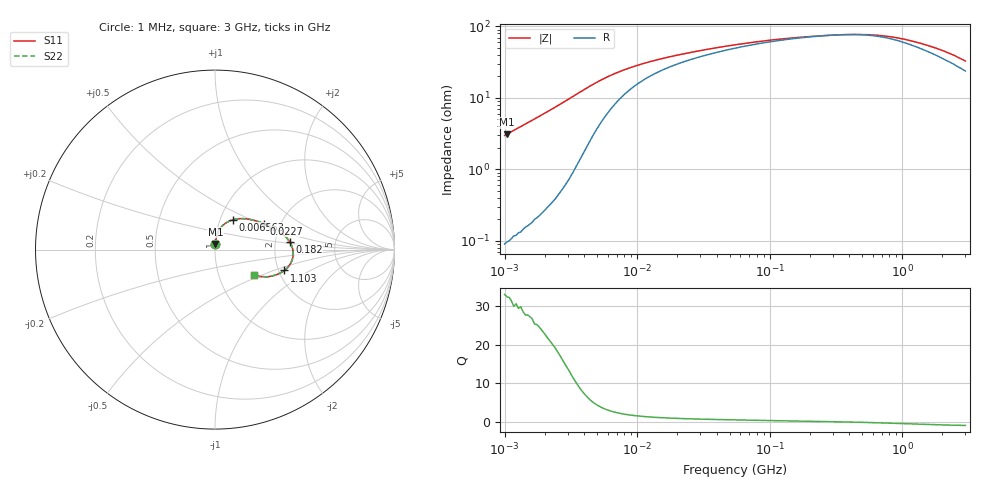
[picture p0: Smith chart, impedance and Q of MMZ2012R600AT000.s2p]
! S-parameter Generated by TDK Corporation
! Copyright(C) 2016 TDK Corporation.
! All Rights Reserved.
! TDK P/N: MMZ2012R600AT000 (Chip Beads)
! Property: |Z|=60¶ at 100MHz
! Size(LxWxT): 2x1.25x0.85mm, 0.079x0.049x0.033inches
! Model Type: s2p (Touchstone File Format Version 1.0)
! Frequency: DC=Yes Start=1MHz Stop=3000MHz 202points Log-sweep
! Note: This model was converted from impedance.
! Model Generated on May. 16, 2016
! Hash(MD5):
! Port Assignments:
!  1 ---@@@--- 2
! Applicable Conditions:
!  Temperature = 25 degC
!  DC Bias Current = 0 A
!  Small Signal Operation
! Terms and conditions regarding TDK Simulation Models
! (1)This simulation model is being provided solely for informational purposes. Please refer to the specifications of the products in terms of detailed characteristics of such products.
! (2)In no event shall TDK Corporation of any of its subsidiaries be liable for any loss or damage arising, directly or indirectly,
!  From any information contained in this simulation model, including, but not limited to loss or damages arising from any inaccuracies, omissions or errors in connection with such information.
! (3)Any and all copyrights on this simulation model are owned by TDK Corporation.
!  Duplication or redistribution of this simulation model without prior written permission from TDK Corporation is prohibited.
! (4)This simulation model is subject to any modification or change without any prior notice.
! (5)Neither TDK Corporation nor any of its subsidiaries shall make any warranty, express or implied,
!  Including but not limited to the correctness, implied warranties of merchantability and fitness for a particular purpose with respect to this simulation models.
! (6)The use of this simulation model shall be deemed to have consented to the terms and conditions hereof.
# MHz S MA R 50
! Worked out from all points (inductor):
!   201 points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, 1 MHz to 3 GHz, reference 50 ohm
!   read as one part in series: L = 477 nH near 1.041 MHz
!   highest Q = 32.5 at 1.041 MHz (marker M1), where L = 476 nH
!   self-resonance near 345.4 MHz
!   S11 on the Smith chart (normalised r, x): 1 MHz: 1.00, +0.06; 6.563 MHz: 1.15, +0.40; 22.7 MHz: 1.64, +0.53; 182 MHz: 2.40, +0.25; 1.103 GHz: 2.15, -0.60; 3 GHz: 1.48, -0.45
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1  0.02985 86.6  0.9987 -1.7  0.9987 -1.7  0.02985 86.6
1.040844  0.03111 86.5  0.9986 -1.8  0.9986 -1.8  0.03111 86.5
2.13957  0.06497 83.6  0.9949 -3.7  0.9949 -3.7  0.06497 83.6
3.067588  0.09602 80.2  0.9882 -5.5  0.9882 -5.5  0.09602 80.2
3.900413  0.1248 75.5  0.9762 -7.1  0.9762 -7.1  0.1248 75.5
5.161903  0.1633 67.0  0.9482 -9.1  0.9482 -9.1  0.1633 67.0
6.563319  0.1951 58.6  0.9138 -10.5  0.9138 -10.5  0.1951 58.6
9.410094  0.2357 47.0  0.8566 -11.6  0.8566 -11.6  0.2357 47.0
14.61624  0.2754 35.9  0.7937 -11.7  0.7937 -11.7  0.2754 35.9
22.70269  0.3086 28.0  0.7417 -11.2  0.7417 -11.2  0.3086 28.0
54.77226  0.3654 17.0  0.6592 -9.3  0.6592 -9.3  0.3654 17.0
99.84923  0.3956 11.2  0.6167 -7.2  0.6167 -7.2  0.3956 11.2
182.0241  0.418 6.0  0.5859 -4.3  0.5859 -4.3  0.418 6.0
213.6344  0.4228 4.6  0.5795 -3.3  0.5795 -3.3  0.4228 4.6
457.0858  0.4366 -3.2  0.5646 2.5  0.5646 2.5  0.4366 -3.2
604.9187  0.4346 -7.0  0.5711 5.3  0.5711 5.3  0.4346 -7.0
800.5644  0.4254 -11.4  0.5889 8.2  0.5889 8.2  0.4254 -11.4
1102.76  0.4036 -16.7  0.6244 10.7  0.6244 10.7  0.4036 -16.7
1519.029  0.3702 -22.2  0.6718 12.0  0.6718 12.0  0.3702 -22.2
1931.433  0.3383 -26.3  0.7126 12.1  0.7126 12.1  0.3383 -26.3
2455.801  0.2999 -30.2  0.7562 11.5  0.7562 11.5  0.2999 -30.2
3000  0.261 -33.2  0.7944 10.4  0.7944 10.4  0.261 -33.2
